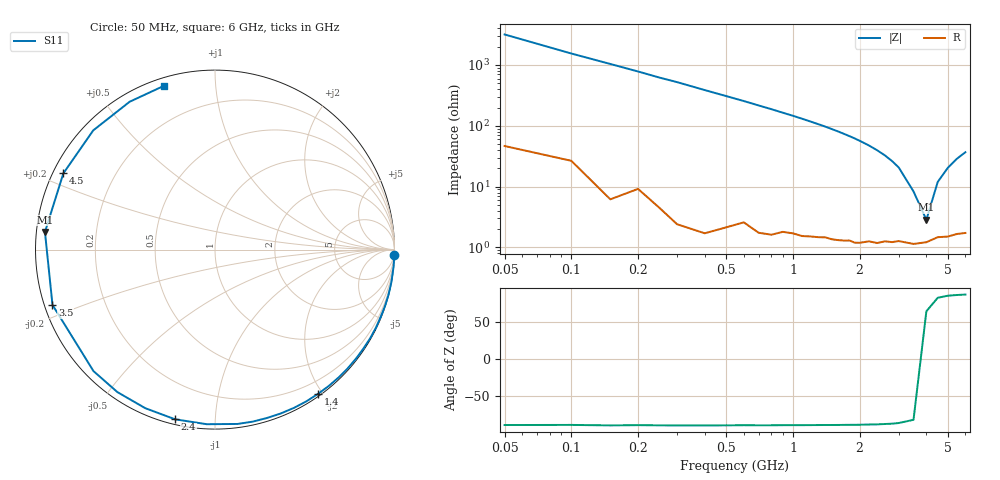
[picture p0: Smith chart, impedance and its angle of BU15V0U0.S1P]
! Infineon Technologies  Discrete & RF Semiconductors
! BB 833
! Si Tuning Diode in SOD323
! VR = 15 V
! S-Parameters:  June  1999
# GHz  S  MA  R  50
!  f  S11
! GHz  MAG  ANG
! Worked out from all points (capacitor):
!   34 points, 50 MHz to 6 GHz, reference 50 ohm
!   read as one part to ground: C = 1.02 pF near 50 MHz
!   lowest |Z| = 2.85 ohm at 4 GHz (marker M1)
!   series resonance near 3.881 GHz, so ESL is about 1.7 nH
!   S11 on the Smith chart (normalised r, x): 50 MHz: 1, -64; 1.4 GHz: 0.03, -1.94; 2.4 GHz: 0.02, -0.79; 3.5 GHz: 0.02, -0.17; 4.5 GHz: 0.03, +0.24; 6 GHz: 0.03, +0.74
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0.05  0.9995 -1.8
0.15  0.9994 -5.5
0.25  0.9989 -9.2
0.4  0.9989 -14.7
0.5  0.9978 -18.4
0.6  0.9962 -22.1
0.8  0.9957 -29.8
1  0.9929 -37.7
1.1  0.9922 -41.8
1.3  0.9894 -50.2
1.4  0.9878 -54.5
1.5  0.9869 -59.0
1.6  0.9855 -63.5
1.7  0.9838 -68.2
1.8  0.9818 -72.9
1.9  0.9813 -77.7
2  0.9794 -82.7
2.2  0.9739 -92.7
2.4  0.9713 -103.2
2.6  0.9652 -113.7
2.8  0.9624 -124.4
3  0.9574 -135.0
3.5  0.9564 -161.2
4  0.9525 174.1
4.5  0.9456 153.3
5  0.9495 135.6
5.5  0.9512 120.0
6  0.9561 107.2
